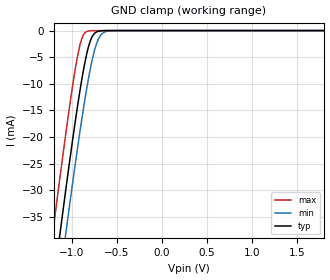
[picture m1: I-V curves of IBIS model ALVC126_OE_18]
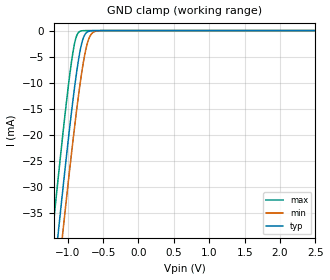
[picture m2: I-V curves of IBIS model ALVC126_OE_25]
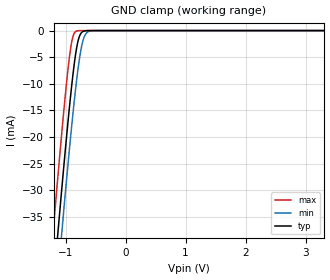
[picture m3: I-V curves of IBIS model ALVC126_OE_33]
| TEXAS INSTRUMENTS INCORPORATED
| Standard Linear and Logic Group
| IBIS Model of SN74ALVC126
| QUADRUPLE BUS BUFFER GATE WITH 3-STATE OUTPUTS
| This file contains package information for the following:
|  SOIC 14-pin (D) package as [Component] ALVC126_D
|  TVSOP 14-pin (DGV) package as [Component] ALVC126_DGV
|  SOP 14-pin (NS) package as [Component] ALVC126_NS
|  TSSOP 14-pin (PW) package as [Component] ALVC126_PW
| This device can be powered at the following Vccs:
|  1.8 volt Vcc
|  2.5 volt Vcc
|  3.3 volt Vcc
| This file provides unique models under the [Model Selector] for each Vcc.
| For operation at a specific Vcc, select the appropriate model after each
| [Model Selector] keyword.
[IBIS Ver]   3.2
[Comment char]  |_char
[File Name]   sn74alvc126.ibs
[File Rev]   1.1 | x_die
[Date]   May 10, 2002
[Source]   Data created from TI-SPICE simulations at TI-SLL.
[Notes]   The following is an IBIS list for the ALVC126.
   Please contact sllibis@ti.com with questions and
   comments concerning SLL IBIS models.
   - We ommitted some Pwr_Clamp data from the input model
   as there is no Power clamp diode at the input
[Disclaimer] Property of Texas Instruments Incorporated.  Unauthorized
   reproduction and/or distribution is strictly prohibited.
   This product is protected under copyright law.
   Created  2002, (C) Copyright  2002, Texas Instruments
   Incorporated, All Rights Reserved
   UNLESS THERE IS A SIGNED, WRITTEN AGREEMENT TO THE
   CONTRARY, TEXAS INSTRUMENTS (TI) IS PROVIDING THE IBIS
   MODELS  AND WITHOUT ANY WARRANTY, EXPRESSED OR
   IMPLIED.  TI assumes no liability for:
   1) the accuracy of the IBIS models provided to your
   company;
   2) the proper functioning of these IBIS Models in your
   design or for any resulting applications; or
   3) infringement of patents, copyrights or intellectual
   property rights resulting from your use of these IBIS
   models.
   TI provides IBIS Models as a service to our customers.
   You and your company shall not distribute, sell or give
   these models to anyone else without prior written
   permission from TI.
   TI reserves the right to make changes to our products or
   to discontinue any semiconductor product or service
   without notice, and advises our customers to obtain the
   latest version of relevant information to verify, before
   placing orders, that the information being relied on is
   current.
   Please be aware that your receipt and use of the IBIS
   information provided shall serve as acceptance of these
   terms and conditions.  If you do not accept these terms,
   you should return or destroy the IBIS models and any
   other accompanying information immediately.
| Component ALVC126_D 14-pin SOIC
[Component]   ALVC126_D
[Manufacturer]   Texas Instruments, Inc.
[Package]
|   typ   min   max
R_pkg   3.100e-02   2.800e-02   3.400e-02
L_pkg   3.109e-09   2.462e-09   3.889e-09
C_pkg   4.730e-13   3.630e-13   6.280e-13
[Pin]   signal_name   model_name   R_pin   L_pin   C_pin
1   1OE   ALVC126_OE   3.300e-02   3.854e-09   6.220e-13
2   1A   ALVC126_IN   3.200e-02   3.188e-09   4.730e-13
3   1Y   ALVC126_OUT   2.800e-02   2.462e-09   3.770e-13
4   2OE   ALVC126_OE   3.100e-02   2.596e-09   3.630e-13
5   2A   ALVC126_IN   2.800e-02   2.521e-09   3.720e-13
6   2Y   ALVC126_OUT   3.400e-02   3.250e-09   4.760e-13
7   GND   GND   3.400e-02   3.889e-09   6.280e-13
8   3Y   ALVC126_OUT   3.400e-02   3.889e-09   6.280e-13
9   3A   ALVC126_IN   3.400e-02   3.250e-09   4.760e-13
10   3OE   ALVC126_OE   2.800e-02   2.521e-09   3.720e-13
11   4Y   ALVC126_OUT   3.100e-02   2.596e-09   3.640e-13
12   4A   ALVC126_IN   2.800e-02   2.462e-09   3.770e-13
13   4OE   ALVC126_OE   3.200e-02   3.188e-09   4.730e-13
14   VCC   POWER   3.300e-02   3.854e-09   6.220e-13
| Component ALVC126_DGV 14-pin TVSOP
[Component]   ALVC126_DGV
[Manufacturer]   Texas Instruments, Inc.
[Package]
|   typ   min   max
R_pkg   3.500e-02   2.000e-02   4.500e-02
L_pkg   2.499e-09   2.077e-09   2.966e-09
C_pkg   3.610e-13   3.050e-13   4.160e-13
[Pin]   signal_name   model_name   R_pin   L_pin   C_pin
1   1OE   ALVC126_OE   2.700e-02   2.717e-09   3.730e-13
2   1A   ALVC126_IN   3.700e-02   2.434e-09   3.980e-13
3   1Y   ALVC126_OUT   3.400e-02   2.200e-09   3.160e-13
4   2OE   ALVC126_OE   2.000e-02   2.077e-09   3.090e-13
5   2A   ALVC126_IN   3.000e-02   2.147e-09   3.050e-13
6   2Y   ALVC126_OUT   4.200e-02   2.580e-09   4.080e-13
7   GND   GND   3.900e-02   2.921e-09   3.850e-13
8   3Y   ALVC126_OUT   3.300e-02   2.841e-09   3.800e-13
9   3A   ALVC126_IN   4.200e-02   2.611e-09   4.100e-13
10   3OE   ALVC126_OE   3.800e-02   2.331e-09   3.290e-13
11   4Y   ALVC126_OUT   2.600e-02   2.223e-09   3.190e-13
12   4A   ALVC126_IN   3.400e-02   2.259e-09   3.130e-13
13   4OE   ALVC126_OE   4.500e-02   2.681e-09   4.160e-13
14   VCC   POWER   4.200e-02   2.966e-09   3.860e-13
| Component ALVC126_NS 14-pin SOP
[Component]   ALVC126_NS
[Manufacturer]   Texas Instruments, Inc.
[Package]
|   typ   min   max
R_pkg   4.500e-02   3.900e-02   5.400e-02
L_pkg   3.796e-09   2.561e-09   4.952e-09
C_pkg   5.280e-13   2.880e-13   7.100e-13
[Pin]   signal_name   model_name   R_pin   L_pin   C_pin
1   1OE   ALVC126_OE   4.700e-02   4.867e-09   7.060e-13
2   1A   ALVC126_IN   5.100e-02   4.083e-09   5.920e-13
3   1Y   ALVC126_OUT   4.100e-02   2.915e-09   3.760e-13
4   2OE   ALVC126_OE   3.900e-02   2.561e-09   2.880e-13
5   2A   ALVC126_IN   4.100e-02   3.101e-09   4.300e-13
6   2Y   ALVC126_OUT   4.700e-02   4.047e-09   5.890e-13
7   GND   GND   5.100e-02   4.909e-09   7.000e-13
8   3Y   ALVC126_OUT   4.500e-02   4.784e-09   6.940e-13
9   3A   ALVC126_IN   5.400e-02   4.176e-09   5.970e-13
10   3OE   ALVC126_OE   3.900e-02   3.287e-09   4.490e-13
11   4Y   ALVC126_OUT   3.900e-02   2.586e-09   2.940e-13
12   4A   ALVC126_IN   4.000e-02   2.802e-09   3.710e-13
13   4OE   ALVC126_OE   4.900e-02   4.080e-09   5.930e-13
14   VCC   POWER   5.200e-02   4.952e-09   7.100e-13
| Component ALVC126_PW 14-pin TSSOP
[Component]   ALVC126_PW
[Manufacturer]   Texas Instruments, Inc.
[Package]
|   typ   min   max
R_pkg   3.200e-02   2.900e-02   3.500e-02
L_pkg   2.378e-09   2.170e-09   2.680e-09
C_pkg   3.140e-13   2.700e-13   3.350e-13
[Pin]   signal_name   model_name   R_pin   L_pin   C_pin
1   1OE   ALVC126_OE   3.300e-02   2.618e-09   3.300e-13
2   1A   ALVC126_IN   3.100e-02   2.313e-09   3.170e-13
3   1Y   ALVC126_OUT   3.000e-02   2.310e-09   3.140e-13
4   2OE   ALVC126_OE   3.100e-02   2.173e-09   2.720e-13
5   2A   ALVC126_IN   3.000e-02   2.204e-09   3.090e-13
6   2Y   ALVC126_OUT   3.200e-02   2.315e-09   3.170e-13
7   GND   GND   3.500e-02   2.680e-09   3.350e-13
8   3Y   ALVC126_OUT   3.300e-02   2.640e-09   3.330e-13
9   3A   ALVC126_IN   3.400e-02   2.347e-09   3.190e-13
10   3OE   ALVC126_OE   2.900e-02   2.277e-09   3.130e-13
11   4Y   ALVC126_OUT   3.100e-02   2.170e-09   2.700e-13
12   4A   ALVC126_IN   3.100e-02   2.244e-09   3.110e-13
13   4OE   ALVC126_OE   3.300e-02   2.343e-09   3.210e-13
14   VCC   POWER   3.500e-02   2.657e-09   3.320e-13
| Model ALVC126_OE
[Model Selector]   ALVC126_OE
ALVC126_OE_18   1.8 volt Vcc
ALVC126_OE_25   2.5 volt Vcc
ALVC126_OE_33   3.3 volt Vcc
| Model ALVC126_IN
[Model Selector]   ALVC126_IN
ALVC126_IN_18   1.8 volt Vcc
ALVC126_IN_25   2.5 volt Vcc
ALVC126_IN_33   3.3 volt Vcc
| Model ALVC126_OUT
[Model Selector]   ALVC126_OUT
ALVC126_OUT_18   1.8 volt Vcc
ALVC126_OUT_25   2.5 volt Vcc
ALVC126_OUT_33   3.3 volt Vcc
| Models and submodels in the file (9): ALVC126_OE_18 (Input), ALVC126_OE_25 (Input), ALVC126_OE_33 (Input), ALVC126_IN_18 (Input), ALVC126_IN_25 (Input), ALVC126_IN_33 (Input), ALVC126_OUT_18 (3-state), ALVC126_OUT_25 (3-state), ALVC126_OUT_33 (3-state)
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[Model]   ALVC126_OE_18
Model_type  Input
Vinl=0.5775
Vinh=1.2675
| variable   typ   min   max
C_comp   3.35pF   2.86pF   4.23pF
[Temperature Range]   40   100   -40
| Ambient temperature   25   85   -40
[Voltage range]   1.8   1.65   1.95
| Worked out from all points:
|   GND clamp passes 1 mA (typ) near -0.77 V on its own axis
[GND Clamp]
| ALVC126_OE_18
|   Voltage   I(typ)   I(min)   I(max)
-1.8V     -129.8mA   -137.8mA   -119.7mA
-1.205V   -48.27mA   -56.56mA   -37.63mA
-1.125V   -37.77mA   -46.06mA   -27.13mA
-1.06V    -29.44mA   -37.69mA   -18.89mA
-980mV    -19.61mA   -27.69mA   -9.485mA
-925mV    -13.29mA   -21.11mA   -4.122mA
-880mV    -8.606mA   -15.99mA   -1.263mA
-835mV    -4.656mA   -11.25mA   -214.1uA
-780mV    -1.472mA   -6.227mA   -17.15uA
-725mV    -285.9uA   -2.596mA   -1.294uA
-615mV    -6.479uA   -167.8uA   -7.303nA
1.8V      1.803pA    4.221pA    1.8pA
[Model]   ALVC126_OE_25
Model_type  Input
Vinl=0.7
Vinh=1.7
| variable   typ   min   max
C_comp   3.29pF   2.69pF   4.23pF
[Temperature Range]   40   100   -40
| Ambient temperature   25   85   -40
[Voltage range]   2.5   2.3   2.7
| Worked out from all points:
|   GND clamp passes 1 mA (typ) near -0.77 V on its own axis
[GND Clamp]
| ALVC126_OE_25
|   Voltage   I(typ)   I(min)   I(max)
-2.5V     -228.1mA   -235.8mA   -218.5mA
-1.23V    -51.59mA   -59.87mA   -40.97mA
-1.2V     -47.61mA   -55.9mA    -36.97mA
-1.13V    -38.42mA   -46.71mA   -27.77mA
-1.07V    -30.71mA   -38.96mA   -20.13mA
-925mV    -13.29mA   -21.11mA   -4.122mA
-880mV    -8.606mA   -15.99mA   -1.263mA
-830mV    -4.281mA   -10.75mA   -171.6uA
-780mV    -1.472mA   -6.227mA   -17.15uA
-720mV    -242.5uA   -2.354mA   -1.023uA
-600mV    -3.832uA   -109.2uA   -3.605nA
2.5V      2.503pA    4.921pA    2.5pA
[Model]   ALVC126_OE_33
Model_type  Input
Vinl=0.8
Vinh=2.0
| variable   typ   min   max
C_comp   3.21pF   2.56pF   4.14pF
[Temperature Range]   40   100   -40
| Ambient temperature   25   85   -40
[Voltage range]   3.3   3   3.6
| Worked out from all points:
|   GND clamp passes 1 mA (typ) near -0.77 V on its own axis
[GND Clamp]
| ALVC126_OE_33
|   Voltage   I(typ)   I(min)   I(max)
-3.3V     -341.5mA   -348.9mA   -332.3mA
-1.215V   -49.6mA    -57.88mA   -38.96mA
-1.185V   -45.62mA   -53.91mA   -34.98mA
-1.125V   -37.77mA   -46.06mA   -27.13mA
-1.065V   -30.08mA   -38.33mA   -19.51mA
-920mV    -12.75mA   -20.53mA   -3.718mA
-875mV    -8.124mA   -15.45mA   -1.065mA
-825mV    -3.922mA   -10.26mA   -137.1uA
-775mV    -1.291mA   -5.83mA    -13.57uA
-715mV    -205.4uA   -2.128mA   -808.5nA
-585mV    -2.266uA   -70.82uA   -1.779nA
3.3V      3.303pA    5.721pA    3.3pA
